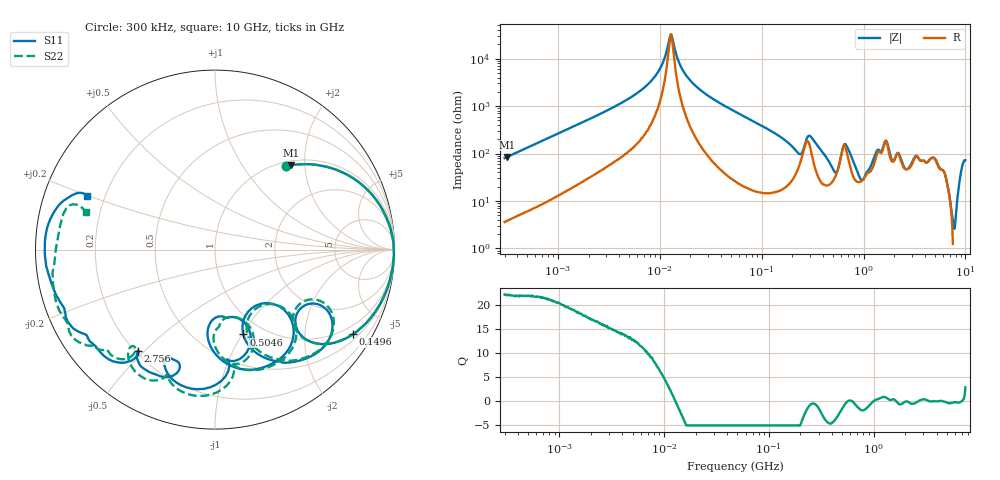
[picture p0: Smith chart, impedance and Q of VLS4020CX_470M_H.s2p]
! S-Parameter Data Generated by TDK Corporation
! Copyright(C) 2024 TDK Corporation.
! All Rights Reserved.
! TDK P/N: VLS4020CX-470M-H (SMD / SMT Inductor (Coil))
! Property: L=47uH at 1MHz
! Size(LxWxT): 4x4x2mm
! Model Type: s2p (Touchstone File Format Version 1.0)
! Frequency: DC=Yes Start=0.3MHz Stop=10000MHz 802points Log-sweep
! Model Generated on May 28, 2024
! Terms and conditions regarding TDK Simulation Models:
! 1)This simulation model is being provided solely for informational
!  purposes. Please refer to the specifications of the products in
!  terms of detailed characteristics of such products.
! 2)In no event shall TDK Corporation of any of its subsidiaries be
!  liable for any loss or damage arising, directly or indirectly,
!  from any information contained in this simulation model, including,
!  but not limited to loss or damages arising from any inaccuracies,
!  omissions or errors in connection with such information.
! 3)Any and all copyrights on this simulation model are owned by
!  TDK Corporation.  Duplication or redistribution of this simulation
!  model without prior written permission from TDK Corporation
!  is prohibited.
! 4)This simulation model is subject to any modification or change
!  without any prior notice.
! 5)Neither TDK Corporation nor any of its subsidiaries shall make any
!  warranty, express or implied, including but not limited to the
!  correctness, implied warranties of merchantability and fitness for
!  a particular purpose with respect to this simulation models.
! 6)The use of this simulation model shall be deemed to have consented
!  to the terms and conditions hereof.
! Port Assignments:
!  1 ---@@@--- 2
! Applicable Conditions:
!  Temperature = 25 degC
!  DC Bias Current = 0 A
!  Small Signal Operation
# Hz S MA R 50
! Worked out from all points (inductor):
!   801 points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, 300 kHz to 10 GHz, reference 50 ohm
!   read as one part in series: L = 42.3 uH near 318.3 kHz
!   highest Q = 22.2 at 318.3 kHz (marker M1), where L = 42.5 uH
!   self-resonance near 12.73 MHz
!   S11 on the Smith chart (normalised r, x): 300 kHz: 1.08, +1.60; 149.6 MHz: 0.67, -3.43; 504.6 MHz: 0.81, -1.01; 2.756 GHz: 0.21, -0.48; 10 GHz: 0.13, +0.20
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300000  0.6117 49.6  0.7637 -37.8  0.7639 -37.8  0.6119 49.6
318337  0.6333 48.0  0.7456 -39.4  0.7456 -39.4  0.6334 48.0
1713600  0.9644 12.3  0.2161 -74.5  0.2161 -74.5  0.9644 12.3
5354396  0.9931 3.2  0.06246 -82.2  0.06242 -82.2  0.993 3.2
9671944  0.9965 0.4  0.01872 -79.1  0.01872 -79.2  0.9964 0.4
1.306337e7  0.9969 -0.9  0.003189 15.3  0.003195 15.3  0.997 -0.9
2.036513e7  0.9965 -3.0  0.03031 81.3  0.03032 81.2  0.9966 -3.0
5.477226e7  0.9874 -10.9  0.128 77.2  0.1281 77.2  0.9874 -10.8
1.495617e8  0.9028 -31.4  0.3732 54.7  0.3732 54.7  0.9019 -31.3
2.351426e8  0.6062 -42.4  0.5442 15.7  0.5443 15.7  0.5913 -42.6
3.126428e8  0.8112 -39.4  0.3476 28.4  0.3476 28.4  0.8072 -37.5
5.046115e8  0.4987 -71.5  0.6839 -3.3  0.6839 -3.3  0.5065 -69.0
5.82867e8  0.4159 -45.7  0.5805 -28.5  0.5805 -28.5  0.4314 -44.6
6.490631e8  0.6607 -48.9  0.352 -22.0  0.352 -22.0  0.671 -47.8
8.987251e8  0.5432 -92.4  0.6477 -21.4  0.6478 -21.4  0.5651 -88.7
1.196827e9  0.396 -72.8  0.6004 -62.9  0.6004 -62.9  0.3884 -74.6
1.35547e9  0.5985 -72.8  0.3899 -79.1  0.39 -79.1  0.6035 -70.1
1.767019e9  0.7789 -104.1  0.2464 -54.8  0.2464 -54.9  0.8204 -99.8
2.756092e9  0.7119 -127.3  0.3202 -91.8  0.3202 -91.9  0.71 -130.7
5.099159e9  0.9113 -153.1  0.08148 -114.4  0.08151 -114.5  0.9312 -147.9
7.763894e9  0.9487 177.4  0.06936 -128.6  0.06933 -128.7  0.8874 -179.7
1e10  0.7754 157.2  0.04918 -126.3  0.04909 -126.4  0.7491 163.9
